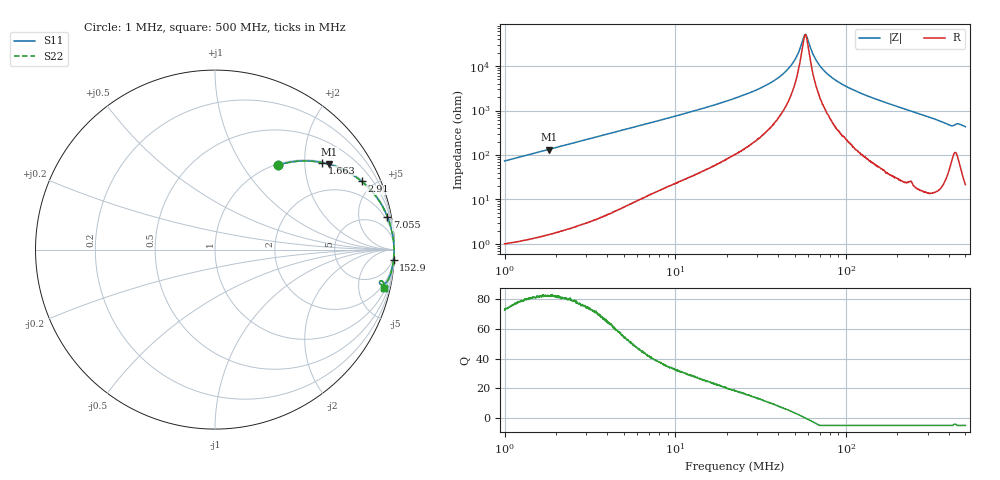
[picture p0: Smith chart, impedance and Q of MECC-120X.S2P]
!s-Parameter Generated by FASTRON Sdn. Bhd.
!FASTRON P/N : MECC-120X
!Keysight Technologies,E4991B,MY54100416,A.01.15
!Date: Mon Mar 16 15:27:24 2026
!Version  : Rev00 Mon Mar 16 15:27:24 2026
!Data & Calibration Information:
!PortZ  Port1:50+j0  Port2:50+j0
!When reading, reference impedance value at option line is always used.
! Remarks : This data is being provided solely for informational purposes.
!Freq	S11	S21	S12	S22
# Hz S dB R 50
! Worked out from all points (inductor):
!   1601 points, 1 MHz to 500 MHz, reference 50 ohm
!   read as one part in series: L = 11.7 uH near 1.032 MHz
!   highest Q = 82.5 at 1.812 MHz (marker M1), where L = 11.7 uH
!   self-resonance near 57.69 MHz
!   S11 on the Smith chart (normalised r, x): 1 MHz: 1.02, +1.47; 1.663 MHz: 1.03, +2.44; 2.91 MHz: 1.06, +4.26; 7.055 MHz: 1, +10; 152.9 MHz: 2, -35; 500 MHz: 1.43, -8.63
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1000000  -4.63 53.3  -1.92 -36.0  -1.92 -36.0  -4.63 53.3
1663329  -2.29 39.1  -4.00 -50.2  -4.00 -50.2  -2.29 39.1
1811711  -2.00 36.8  -4.46 -52.6  -4.46 -52.6  -2.00 36.8
2820919  -0.96 25.7  -7.26 -63.6  -7.26 -63.6  -0.96 25.7
2909950  -0.91 25.0  -7.48 -64.3  -7.48 -64.3  -0.91 25.0
7054865  -0.20 10.8  -14.54 -77.8  -14.54 -77.8  -0.20 10.8
7957584  -0.16 9.6  -15.58 -78.9  -15.58 -78.9  -0.16 9.6
2.236068e7  -0.04 3.0  -25.54 -83.8  -25.54 -83.8  -0.04 3.0
3.323107e7  -0.02 1.6  -30.98 -83.4  -30.98 -83.4  -0.02 1.6
4.2775e7  -0.02 0.8  -36.52 -80.8  -36.52 -80.8  -0.02 0.8
4.996481e7  -0.02 0.4  -42.66 -73.5  -42.66 -73.5  -0.02 0.4
5.746337e7  -0.02 0.0  -54.02 -7.2  -54.02 -7.2  -0.02 0.0
5.927696e7  -0.02 -0.1  -52.65 33.1  -52.65 33.1  -0.02 -0.1
6.307767e7  -0.02 -0.2  -46.53 65.5  -46.53 65.5  -0.02 -0.2
7.059833e7  -0.02 -0.6  -39.89 78.7  -39.89 78.7  -0.02 -0.6
8.343135e7  -0.02 -1.1  -34.59 83.4  -34.59 83.4  -0.02 -1.1
1.065617e8  -0.02 -1.9  -29.81 84.9  -29.81 84.9  -0.02 -1.9
1.529251e8  -0.03 -3.3  -24.88 84.9  -24.88 84.9  -0.03 -3.3
1.77937e8  -0.04 -4.0  -23.12 84.5  -23.12 84.5  -0.04 -4.0
4.006999e8  -0.35 -11.6  -13.86 73.0  -13.86 73.0  -0.35 -11.6
4.519722e8  -0.44 -10.7  -14.47 69.4  -14.47 69.4  -0.44 -10.7
5e8  -0.32 -12.9  -13.03 74.3  -13.03 74.3  -0.32 -12.9
